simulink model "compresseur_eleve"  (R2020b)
settings: Solver=VariableStepAuto  StartTime=0.0  StopTime=1  RelTol=1e-3
PreLoadFcn:
  | compresseur_7_DataFile
model workspace: external: MATLAB File (data not in the file)
undefined symbols (not defined in the file or in its folder): deg, kg, m, mm, N, s, smiData, X, Y, Z
libraries: sm_lib x91, fl_lib x8, nesl_utility x5, ee_lib x1
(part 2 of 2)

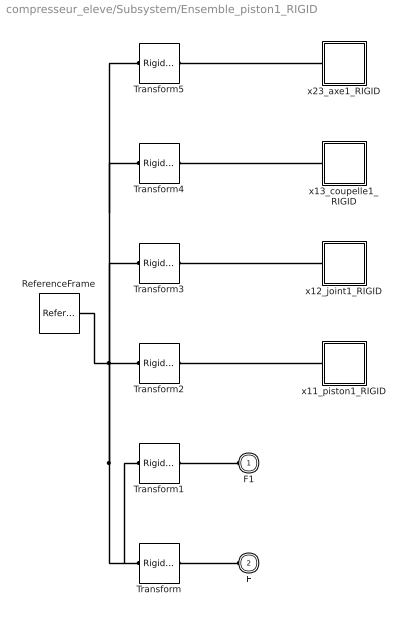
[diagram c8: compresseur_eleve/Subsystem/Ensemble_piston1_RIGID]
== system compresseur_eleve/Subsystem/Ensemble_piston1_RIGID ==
  ReferenceFrame : sm_lib/Frames and Transforms/Reference Frame
  Transform : sm_lib/Frames and Transforms/Rigid Transform  TranslationMethod=Cartesian  TranslationStandardOffset=0  TranslationLengthUnit=mm  TranslationStandardAxis=+Z  TranslationCartesianOffset=smiData.RigidTransform(2).translation  TranslationROffset=0  TranslationROffsetUnits=m  TranslationZOffset=0  TranslationZOffsetUnits=m  TranslationThetaOffset=0  TranslationThetaOffsetUnits=deg  RotationMethod=ArbitraryAxis  RotationAngleUnits=rad  RotationStandardAxis=+Z  RotationAngle=smiData.RigidTransform(2).angle  RotationArbitraryAxis=smiData.RigidTransform(2).axis  FollAlignAxisA=+X  BaseAlignAxisA=+Y  FollAlignAxisB=+Y  BaseAlignAxisB=+Z  RotationSequenceAxes=FollowerAxes  RotationSequence=XYX  RotationSequenceAngles=[0 0 0]  RotationSequenceAnglesUnits=deg  RotationMatrix=[1 0 0; 0 1 0; 0 0 1]
  Transform1 : sm_lib/Frames and Transforms/Rigid Transform  TranslationMethod=Cartesian  TranslationStandardOffset=0  TranslationLengthUnit=mm  TranslationStandardAxis=+Z  TranslationCartesianOffset=smiData.RigidTransform(6).translation  TranslationROffset=0  TranslationROffsetUnits=m  TranslationZOffset=0  TranslationZOffsetUnits=m  TranslationThetaOffset=0  TranslationThetaOffsetUnits=deg  RotationMethod=ArbitraryAxis  RotationAngleUnits=rad  RotationStandardAxis=+Z  RotationAngle=smiData.RigidTransform(6).angle  RotationArbitraryAxis=smiData.RigidTransform(6).axis  FollAlignAxisA=+X  BaseAlignAxisA=+Y  FollAlignAxisB=+Y  BaseAlignAxisB=+Z  RotationSequenceAxes=FollowerAxes  RotationSequence=XYX  RotationSequenceAngles=[0 0 0]  RotationSequenceAnglesUnits=deg  RotationMatrix=[1 0 0; 0 1 0; 0 0 1]
  Transform2 : sm_lib/Frames and Transforms/Rigid Transform  TranslationMethod=Cartesian  TranslationStandardOffset=0  TranslationLengthUnit=mm  TranslationStandardAxis=+Z  TranslationCartesianOffset=smiData.RigidTransform(21).translation  TranslationROffset=0  TranslationROffsetUnits=m  TranslationZOffset=0  TranslationZOffsetUnits=m  TranslationThetaOffset=0  TranslationThetaOffsetUnits=deg  RotationMethod=ArbitraryAxis  RotationAngleUnits=rad  RotationStandardAxis=+Z  RotationAngle=smiData.RigidTransform(21).angle  RotationArbitraryAxis=smiData.RigidTransform(21).axis  FollAlignAxisA=+X  BaseAlignAxisA=+Y  FollAlignAxisB=+Y  BaseAlignAxisB=+Z  RotationSequenceAxes=FollowerAxes  RotationSequence=XYX  RotationSequenceAngles=[0 0 0]  RotationSequenceAnglesUnits=deg  RotationMatrix=[1 0 0; 0 1 0; 0 0 1]
  Transform3 : sm_lib/Frames and Transforms/Rigid Transform  TranslationMethod=Cartesian  TranslationStandardOffset=0  TranslationLengthUnit=mm  TranslationStandardAxis=+Z  TranslationCartesianOffset=smiData.RigidTransform(22).translation  TranslationROffset=0  TranslationROffsetUnits=m  TranslationZOffset=0  TranslationZOffsetUnits=m  TranslationThetaOffset=0  TranslationThetaOffsetUnits=deg  RotationMethod=ArbitraryAxis  RotationAngleUnits=rad  RotationStandardAxis=+Z  RotationAngle=smiData.RigidTransform(22).angle  RotationArbitraryAxis=smiData.RigidTransform(22).axis  FollAlignAxisA=+X  BaseAlignAxisA=+Y  FollAlignAxisB=+Y  BaseAlignAxisB=+Z  RotationSequenceAxes=FollowerAxes  RotationSequence=XYX  RotationSequenceAngles=[0 0 0]  RotationSequenceAnglesUnits=deg  RotationMatrix=[1 0 0; 0 1 0; 0 0 1]
  Transform4 : sm_lib/Frames and Transforms/Rigid Transform  TranslationMethod=Cartesian  TranslationStandardOffset=0  TranslationLengthUnit=mm  TranslationStandardAxis=+Z  TranslationCartesianOffset=smiData.RigidTransform(23).translation  TranslationROffset=0  TranslationROffsetUnits=m  TranslationZOffset=0  TranslationZOffsetUnits=m  TranslationThetaOffset=0  TranslationThetaOffsetUnits=deg  RotationMethod=ArbitraryAxis  RotationAngleUnits=rad  RotationStandardAxis=+Z  RotationAngle=smiData.RigidTransform(23).angle  RotationArbitraryAxis=smiData.RigidTransform(23).axis  FollAlignAxisA=+X  BaseAlignAxisA=+Y  FollAlignAxisB=+Y  BaseAlignAxisB=+Z  RotationSequenceAxes=FollowerAxes  RotationSequence=XYX  RotationSequenceAngles=[0 0 0]  RotationSequenceAnglesUnits=deg  RotationMatrix=[1 0 0; 0 1 0; 0 0 1]
  Transform5 : sm_lib/Frames and Transforms/Rigid Transform  TranslationMethod=Cartesian  TranslationStandardOffset=0  TranslationLengthUnit=mm  TranslationStandardAxis=+Z  TranslationCartesianOffset=smiData.RigidTransform(24).translation  TranslationROffset=0  TranslationROffsetUnits=m  TranslationZOffset=0  TranslationZOffsetUnits=m  TranslationThetaOffset=0  TranslationThetaOffsetUnits=deg  RotationMethod=ArbitraryAxis  RotationAngleUnits=rad  RotationStandardAxis=+Z  RotationAngle=smiData.RigidTransform(24).angle  RotationArbitraryAxis=smiData.RigidTransform(24).axis  FollAlignAxisA=+X  BaseAlignAxisA=+Y  FollAlignAxisB=+Y  BaseAlignAxisB=+Z  RotationSequenceAxes=FollowerAxes  RotationSequence=XYX  RotationSequenceAngles=[0 0 0]  RotationSequenceAnglesUnits=deg  RotationMatrix=[1 0 0; 0 1 0; 0 0 1]
  x11_piston1_RIGID : Subsystem
  x12_joint1_RIGID : Subsystem
  x13_coupelle1_RIGID : Subsystem
  x23_axe1_RIGID : Subsystem
  F1 : PMIOPort  Side=Left
  F : PMIOPort  Port=2  Side=Left
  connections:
  Transform/LConn1 -- ReferenceFrame/RConn1 -- Transform4/LConn1 -- Transform5/LConn1 -- Transform3/LConn1 -- Transform2/LConn1 -- Transform1/LConn1
  Transform/RConn1 -- F/RConn1
  Transform1/RConn1 -- F1/RConn1
  Transform2/RConn1 -- x11_piston1_RIGID/LConn1
  Transform3/RConn1 -- x12_joint1_RIGID/LConn1
  Transform4/RConn1 -- x13_coupelle1_RIGID/LConn1
  Transform5/RConn1 -- x23_axe1_RIGID/LConn1

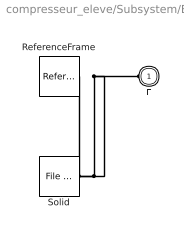
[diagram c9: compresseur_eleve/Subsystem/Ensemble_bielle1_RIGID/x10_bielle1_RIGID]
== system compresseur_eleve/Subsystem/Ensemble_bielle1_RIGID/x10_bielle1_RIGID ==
  ReferenceFrame : sm_lib/Frames and Transforms/Reference Frame
  Solid : sm_lib/Body Elements/File Solid  ExtGeomFileName=10_bielle_ipt_a8871c2b.STL  UnitType=Custom  ExtGeomFileUnits=mm  StepReaderType=HEX  ExportConvexHullGeometry=off  InertiaType=Custom  Mass=smiData.Solid(10).mass  MassUnits=kg  CenterOfMass=smiData.Solid(10).CoM  CenterOfMassUnits=mm  MomentsOfInertia=smiData.Solid(10).MoI  MomentsOfInertiaUnits=kg*mm^2  ProductsOfInertia=smiData.Solid(10).PoI  ProductsOfInertiaUnits=kg*mm^2  BasedOnType=DensityFromFile  Density=1000  DensityUnits=kg/m^3  DoExposeReferenceFrame=on  SerializedFrames=<Frames/>  GraphicType=FromGeometry  MarkerShape=Sphere  MarkerSize=10  GraphicVisPropType=SimpleVisualProperties  GraphicDiffuseColor=smiData.Solid(10).color  GraphicSpecularColor=[0.5 0.5 0.5 1.0]  GraphicAmbientColor=[0.15 0.15 0.15 1.0]  GraphicEmissiveColor=[0.0 0.0 0.0 1.0]  GraphicShininess=75  GraphicOpacity=smiData.Solid(10).opacity
  F : PMIOPort  Side=Left
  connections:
  Solid/RConn1 -- ReferenceFrame/RConn1 -- F/RConn1

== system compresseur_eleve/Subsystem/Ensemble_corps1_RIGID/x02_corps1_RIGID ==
  ReferenceFrame : sm_lib/Frames and Transforms/Reference Frame
  Solid : sm_lib/Body Elements/File Solid  ExtGeomFileName=02_corps_1_ipt_c583bf0c.STL  UnitType=Custom  ExtGeomFileUnits=mm  StepReaderType=HEX  ExportConvexHullGeometry=off  InertiaType=Custom  Mass=smiData.Solid(1).mass  MassUnits=kg  CenterOfMass=smiData.Solid(1).CoM  CenterOfMassUnits=mm  MomentsOfInertia=smiData.Solid(1).MoI  MomentsOfInertiaUnits=kg*mm^2  ProductsOfInertia=smiData.Solid(1).PoI  ProductsOfInertiaUnits=kg*mm^2  BasedOnType=DensityFromFile  Density=1000  DensityUnits=kg/m^3  DoExposeReferenceFrame=on  SerializedFrames=<Frames/>  GraphicType=FromGeometry  MarkerShape=Sphere  MarkerSize=10  GraphicVisPropType=SimpleVisualProperties  GraphicDiffuseColor=smiData.Solid(1).color  GraphicSpecularColor=[0.5 0.5 0.5 1.0]  GraphicAmbientColor=[0.15 0.15 0.15 1.0]  GraphicEmissiveColor=[0.0 0.0 0.0 1.0]  GraphicShininess=75  GraphicOpacity=smiData.Solid(1).opacity
  F : PMIOPort  Side=Left
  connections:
  Solid/RConn1 -- ReferenceFrame/RConn1 -- F/RConn1

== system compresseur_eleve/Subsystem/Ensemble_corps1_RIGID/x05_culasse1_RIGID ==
  ReferenceFrame : sm_lib/Frames and Transforms/Reference Frame
  Solid : sm_lib/Body Elements/File Solid  ExtGeomFileName=05_culasse_1_ipt_d9f37117.STL  UnitType=Custom  ExtGeomFileUnits=mm  StepReaderType=HEX  ExportConvexHullGeometry=off  InertiaType=Custom  Mass=smiData.Solid(2).mass  MassUnits=kg  CenterOfMass=smiData.Solid(2).CoM  CenterOfMassUnits=mm  MomentsOfInertia=smiData.Solid(2).MoI  MomentsOfInertiaUnits=kg*mm^2  ProductsOfInertia=smiData.Solid(2).PoI  ProductsOfInertiaUnits=kg*mm^2  BasedOnType=DensityFromFile  Density=1000  DensityUnits=kg/m^3  DoExposeReferenceFrame=on  SerializedFrames=<Frames/>  GraphicType=FromGeometry  MarkerShape=Sphere  MarkerSize=10  GraphicVisPropType=SimpleVisualProperties  GraphicDiffuseColor=smiData.Solid(2).color  GraphicSpecularColor=[0.5 0.5 0.5 1.0]  GraphicAmbientColor=[0.15 0.15 0.15 1.0]  GraphicEmissiveColor=[0.0 0.0 0.0 1.0]  GraphicShininess=75  GraphicOpacity=smiData.Solid(2).opacity
  F : PMIOPort  Side=Left
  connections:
  Solid/RConn1 -- ReferenceFrame/RConn1 -- F/RConn1

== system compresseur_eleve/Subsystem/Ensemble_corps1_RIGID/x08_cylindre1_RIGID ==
  ReferenceFrame : sm_lib/Frames and Transforms/Reference Frame
  Solid : sm_lib/Body Elements/File Solid  ExtGeomFileName=08_cylindre_1_ipt_a42fec77.STL  UnitType=Custom  ExtGeomFileUnits=mm  StepReaderType=HEX  ExportConvexHullGeometry=off  InertiaType=Custom  Mass=smiData.Solid(3).mass  MassUnits=kg  CenterOfMass=smiData.Solid(3).CoM  CenterOfMassUnits=mm  MomentsOfInertia=smiData.Solid(3).MoI  MomentsOfInertiaUnits=kg*mm^2  ProductsOfInertia=smiData.Solid(3).PoI  ProductsOfInertiaUnits=kg*mm^2  BasedOnType=DensityFromFile  Density=1000  DensityUnits=kg/m^3  DoExposeReferenceFrame=on  SerializedFrames=<Frames/>  GraphicType=FromGeometry  MarkerShape=Sphere  MarkerSize=10  GraphicVisPropType=SimpleVisualProperties  GraphicDiffuseColor=smiData.Solid(3).color  GraphicSpecularColor=[0.5 0.5 0.5 1.0]  GraphicAmbientColor=[0.15 0.15 0.15 1.0]  GraphicEmissiveColor=[0.0 0.0 0.0 1.0]  GraphicShininess=75  GraphicOpacity=smiData.Solid(3).opacity
  F : PMIOPort  Side=Left
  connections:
  Solid/RConn1 -- ReferenceFrame/RConn1 -- F/RConn1

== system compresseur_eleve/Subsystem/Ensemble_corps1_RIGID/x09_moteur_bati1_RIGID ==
  ReferenceFrame : sm_lib/Frames and Transforms/Reference Frame
  Solid : sm_lib/Body Elements/File Solid  ExtGeomFileName=09_moteur_bati_1_ipt_87beb56e.STL  UnitType=Custom  ExtGeomFileUnits=mm  StepReaderType=HEX  ExportConvexHullGeometry=off  InertiaType=Custom  Mass=smiData.Solid(4).mass  MassUnits=kg  CenterOfMass=smiData.Solid(4).CoM  CenterOfMassUnits=mm  MomentsOfInertia=smiData.Solid(4).MoI  MomentsOfInertiaUnits=kg*mm^2  ProductsOfInertia=smiData.Solid(4).PoI  ProductsOfInertiaUnits=kg*mm^2  BasedOnType=DensityFromFile  Density=1000  DensityUnits=kg/m^3  DoExposeReferenceFrame=on  SerializedFrames=<Frames/>  GraphicType=FromGeometry  MarkerShape=Sphere  MarkerSize=10  GraphicVisPropType=SimpleVisualProperties  GraphicDiffuseColor=smiData.Solid(4).color  GraphicSpecularColor=[0.5 0.5 0.5 1.0]  GraphicAmbientColor=[0.15 0.15 0.15 1.0]  GraphicEmissiveColor=[0.0 0.0 0.0 1.0]  GraphicShininess=75  GraphicOpacity=smiData.Solid(4).opacity
  F : PMIOPort  Side=Left
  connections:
  Solid/RConn1 -- ReferenceFrame/RConn1 -- F/RConn1

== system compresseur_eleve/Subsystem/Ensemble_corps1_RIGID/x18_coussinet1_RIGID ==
  ReferenceFrame : sm_lib/Frames and Transforms/Reference Frame
  Solid : sm_lib/Body Elements/File Solid  ExtGeomFileName=18_coussinet_1_ipt_47bc357b.STL  UnitType=Custom  ExtGeomFileUnits=mm  StepReaderType=HEX  ExportConvexHullGeometry=off  InertiaType=Custom  Mass=smiData.Solid(5).mass  MassUnits=kg  CenterOfMass=smiData.Solid(5).CoM  CenterOfMassUnits=mm  MomentsOfInertia=smiData.Solid(5).MoI  MomentsOfInertiaUnits=kg*mm^2  ProductsOfInertia=smiData.Solid(5).PoI  ProductsOfInertiaUnits=kg*mm^2  BasedOnType=DensityFromFile  Density=1000  DensityUnits=kg/m^3  DoExposeReferenceFrame=on  SerializedFrames=<Frames/>  GraphicType=FromGeometry  MarkerShape=Sphere  MarkerSize=10  GraphicVisPropType=SimpleVisualProperties  GraphicDiffuseColor=smiData.Solid(5).color  GraphicSpecularColor=[0.5 0.5 0.5 1.0]  GraphicAmbientColor=[0.15 0.15 0.15 1.0]  GraphicEmissiveColor=[0.0 0.0 0.0 1.0]  GraphicShininess=75  GraphicOpacity=smiData.Solid(5).opacity
  F : PMIOPort  Side=Left
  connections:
  Solid/RConn1 -- ReferenceFrame/RConn1 -- F/RConn1

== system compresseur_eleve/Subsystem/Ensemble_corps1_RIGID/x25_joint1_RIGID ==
  ReferenceFrame : sm_lib/Frames and Transforms/Reference Frame
  Solid : sm_lib/Body Elements/File Solid  ExtGeomFileName=25_joint_1_ipt_2419a34a.STL  UnitType=Custom  ExtGeomFileUnits=mm  StepReaderType=HEX  ExportConvexHullGeometry=off  InertiaType=Custom  Mass=smiData.Solid(6).mass  MassUnits=kg  CenterOfMass=smiData.Solid(6).CoM  CenterOfMassUnits=mm  MomentsOfInertia=smiData.Solid(6).MoI  MomentsOfInertiaUnits=kg*mm^2  ProductsOfInertia=smiData.Solid(6).PoI  ProductsOfInertiaUnits=kg*mm^2  BasedOnType=DensityFromFile  Density=1000  DensityUnits=kg/m^3  DoExposeReferenceFrame=on  SerializedFrames=<Frames/>  GraphicType=FromGeometry  MarkerShape=Sphere  MarkerSize=10  GraphicVisPropType=SimpleVisualProperties  GraphicDiffuseColor=smiData.Solid(6).color  GraphicSpecularColor=[0.5 0.5 0.5 1.0]  GraphicAmbientColor=[0.15 0.15 0.15 1.0]  GraphicEmissiveColor=[0.0 0.0 0.0 1.0]  GraphicShininess=75  GraphicOpacity=smiData.Solid(6).opacity
  F : PMIOPort  Side=Left
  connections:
  Solid/RConn1 -- ReferenceFrame/RConn1 -- F/RConn1

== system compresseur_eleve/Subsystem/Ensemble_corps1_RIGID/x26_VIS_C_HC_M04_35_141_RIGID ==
  ReferenceFrame : sm_lib/Frames and Transforms/Reference Frame
  Solid : sm_lib/Body Elements/File Solid  ExtGeomFileName=26_VIS C HC_ M04-35-14_1_ipt_1f7a07f4.STL  UnitType=Custom  ExtGeomFileUnits=mm  StepReaderType=HEX  ExportConvexHullGeometry=off  InertiaType=Custom  Mass=smiData.Solid(7).mass  MassUnits=kg  CenterOfMass=smiData.Solid(7).CoM  CenterOfMassUnits=mm  MomentsOfInertia=smiData.Solid(7).MoI  MomentsOfInertiaUnits=kg*mm^2  ProductsOfInertia=smiData.Solid(7).PoI  ProductsOfInertiaUnits=kg*mm^2  BasedOnType=DensityFromFile  Density=1000  DensityUnits=kg/m^3  DoExposeReferenceFrame=on  SerializedFrames=<Frames/>  GraphicType=FromGeometry  MarkerShape=Sphere  MarkerSize=10  GraphicVisPropType=SimpleVisualProperties  GraphicDiffuseColor=smiData.Solid(7).color  GraphicSpecularColor=[0.5 0.5 0.5 1.0]  GraphicAmbientColor=[0.15 0.15 0.15 1.0]  GraphicEmissiveColor=[0.0 0.0 0.0 1.0]  GraphicShininess=75  GraphicOpacity=smiData.Solid(7).opacity
  F : PMIOPort  Side=Left
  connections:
  Solid/RConn1 -- ReferenceFrame/RConn1 -- F/RConn1

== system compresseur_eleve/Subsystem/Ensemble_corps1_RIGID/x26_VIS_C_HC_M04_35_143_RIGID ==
  ReferenceFrame : sm_lib/Frames and Transforms/Reference Frame
  Solid : sm_lib/Body Elements/File Solid  ExtGeomFileName=26_VIS C HC_ M04-35-14_ipt_c4dcb1c0.STL  UnitType=Custom  ExtGeomFileUnits=mm  StepReaderType=HEX  ExportConvexHullGeometry=off  InertiaType=Custom  Mass=smiData.Solid(8).mass  MassUnits=kg  CenterOfMass=smiData.Solid(8).CoM  CenterOfMassUnits=mm  MomentsOfInertia=smiData.Solid(8).MoI  MomentsOfInertiaUnits=kg*mm^2  ProductsOfInertia=smiData.Solid(8).PoI  ProductsOfInertiaUnits=kg*mm^2  BasedOnType=DensityFromFile  Density=1000  DensityUnits=kg/m^3  DoExposeReferenceFrame=on  SerializedFrames=<Frames/>  GraphicType=FromGeometry  MarkerShape=Sphere  MarkerSize=10  GraphicVisPropType=SimpleVisualProperties  GraphicDiffuseColor=smiData.Solid(8).color  GraphicSpecularColor=[0.5 0.5 0.5 1.0]  GraphicAmbientColor=[0.15 0.15 0.15 1.0]  GraphicEmissiveColor=[0.0 0.0 0.0 1.0]  GraphicShininess=75  GraphicOpacity=smiData.Solid(8).opacity
  F : PMIOPort  Side=Left
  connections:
  Solid/RConn1 -- ReferenceFrame/RConn1 -- F/RConn1

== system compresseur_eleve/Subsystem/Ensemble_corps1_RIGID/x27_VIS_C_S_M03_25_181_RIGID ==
  ReferenceFrame : sm_lib/Frames and Transforms/Reference Frame
  Solid : sm_lib/Body Elements/File Solid  ExtGeomFileName=27_VIS C S_ M03-25-18_ipt_43eec25f.STL  UnitType=Custom  ExtGeomFileUnits=mm  StepReaderType=HEX  ExportConvexHullGeometry=off  InertiaType=Custom  Mass=smiData.Solid(9).mass  MassUnits=kg  CenterOfMass=smiData.Solid(9).CoM  CenterOfMassUnits=mm  MomentsOfInertia=smiData.Solid(9).MoI  MomentsOfInertiaUnits=kg*mm^2  ProductsOfInertia=smiData.Solid(9).PoI  ProductsOfInertiaUnits=kg*mm^2  BasedOnType=DensityFromFile  Density=1000  DensityUnits=kg/m^3  DoExposeReferenceFrame=on  SerializedFrames=<Frames/>  GraphicType=FromGeometry  MarkerShape=Sphere  MarkerSize=10  GraphicVisPropType=SimpleVisualProperties  GraphicDiffuseColor=smiData.Solid(9).color  GraphicSpecularColor=[0.5 0.5 0.5 1.0]  GraphicAmbientColor=[0.15 0.15 0.15 1.0]  GraphicEmissiveColor=[0.0 0.0 0.0 1.0]  GraphicShininess=75  GraphicOpacity=smiData.Solid(9).opacity
  F : PMIOPort  Side=Left
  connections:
  Solid/RConn1 -- ReferenceFrame/RConn1 -- F/RConn1

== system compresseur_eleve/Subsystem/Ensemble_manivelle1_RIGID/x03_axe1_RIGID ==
  ReferenceFrame : sm_lib/Frames and Transforms/Reference Frame
  Solid : sm_lib/Body Elements/File Solid  ExtGeomFileName=03_axe_ipt_3151f0da.STL  UnitType=Custom  ExtGeomFileUnits=mm  StepReaderType=HEX  ExportConvexHullGeometry=off  InertiaType=Custom  Mass=smiData.Solid(15).mass  MassUnits=kg  CenterOfMass=smiData.Solid(15).CoM  CenterOfMassUnits=mm  MomentsOfInertia=smiData.Solid(15).MoI  MomentsOfInertiaUnits=kg*mm^2  ProductsOfInertia=smiData.Solid(15).PoI  ProductsOfInertiaUnits=kg*mm^2  BasedOnType=DensityFromFile  Density=1000  DensityUnits=kg/m^3  DoExposeReferenceFrame=on  SerializedFrames=<Frames/>  GraphicType=FromGeometry  MarkerShape=Sphere  MarkerSize=10  GraphicVisPropType=SimpleVisualProperties  GraphicDiffuseColor=smiData.Solid(15).color  GraphicSpecularColor=[0.5 0.5 0.5 1.0]  GraphicAmbientColor=[0.15 0.15 0.15 1.0]  GraphicEmissiveColor=[0.0 0.0 0.0 1.0]  GraphicShininess=75  GraphicOpacity=smiData.Solid(15).opacity
  F : PMIOPort  Side=Left
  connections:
  Solid/RConn1 -- ReferenceFrame/RConn1 -- F/RConn1

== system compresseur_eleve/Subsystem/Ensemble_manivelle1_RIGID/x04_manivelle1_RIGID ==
  ReferenceFrame : sm_lib/Frames and Transforms/Reference Frame
  Solid : sm_lib/Body Elements/File Solid  ExtGeomFileName=04_manivelle_ipt_16c0bde3.STL  UnitType=Custom  ExtGeomFileUnits=mm  StepReaderType=HEX  ExportConvexHullGeometry=off  InertiaType=Custom  Mass=smiData.Solid(16).mass  MassUnits=kg  CenterOfMass=smiData.Solid(16).CoM  CenterOfMassUnits=mm  MomentsOfInertia=smiData.Solid(16).MoI  MomentsOfInertiaUnits=kg*mm^2  ProductsOfInertia=smiData.Solid(16).PoI  ProductsOfInertiaUnits=kg*mm^2  BasedOnType=DensityFromFile  Density=1000  DensityUnits=kg/m^3  DoExposeReferenceFrame=on  SerializedFrames=<Frames/>  GraphicType=FromGeometry  MarkerShape=Sphere  MarkerSize=10  GraphicVisPropType=SimpleVisualProperties  GraphicDiffuseColor=smiData.Solid(16).color  GraphicSpecularColor=[0.5 0.5 0.5 1.0]  GraphicAmbientColor=[0.15 0.15 0.15 1.0]  GraphicEmissiveColor=[0.0 0.0 0.0 1.0]  GraphicShininess=75  GraphicOpacity=smiData.Solid(16).opacity
  F : PMIOPort  Side=Left
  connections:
  Solid/RConn1 -- ReferenceFrame/RConn1 -- F/RConn1

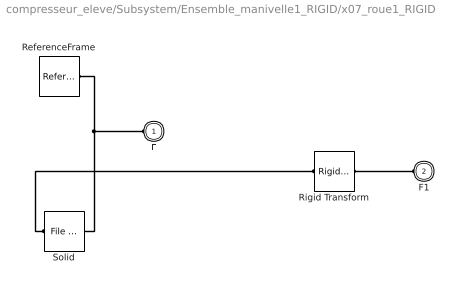
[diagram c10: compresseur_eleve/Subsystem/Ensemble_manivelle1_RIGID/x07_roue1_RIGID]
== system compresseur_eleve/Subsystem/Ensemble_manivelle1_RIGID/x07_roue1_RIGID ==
  ReferenceFrame : sm_lib/Frames and Transforms/Reference Frame
  Rigid Transform : sm_lib/Frames and Transforms/Rigid Transform  TranslationMethod=Cartesian  TranslationStandardOffset=0  TranslationLengthUnit=mm  TranslationStandardAxis=+Z  TranslationCartesianOffset=[0 0 -8]  TranslationROffset=0  TranslationROffsetUnits=m  TranslationZOffset=0  TranslationZOffsetUnits=m  TranslationThetaOffset=0  TranslationThetaOffsetUnits=deg  RotationMethod=None  RotationAngleUnits=deg  RotationStandardAxis=+Z  RotationAngle=0.0  RotationArbitraryAxis=[0 0 1]  FollAlignAxisA=+X  BaseAlignAxisA=+Y  FollAlignAxisB=+Y  BaseAlignAxisB=+Z  RotationSequenceAxes=FollowerAxes  RotationSequence=XYX  RotationSequenceAngles=[0 0 0]  RotationSequenceAnglesUnits=deg  RotationMatrix=[1 0 0; 0 1 0; 0 0 1]
  Solid : sm_lib/Body Elements/File Solid  ExtGeomFileName=07_roue_ipt_2ddf42d4.STL  UnitType=Custom  ExtGeomFileUnits=mm  StepReaderType=HEX  ExportConvexHullGeometry=off  InertiaType=Custom  Mass=smiData.Solid(17).mass  MassUnits=kg  CenterOfMass=smiData.Solid(17).CoM  CenterOfMassUnits=mm  MomentsOfInertia=smiData.Solid(17).MoI  MomentsOfInertiaUnits=kg*mm^2  ProductsOfInertia=smiData.Solid(17).PoI  ProductsOfInertiaUnits=kg*mm^2  BasedOnType=DensityFromFile  Density=1000  DensityUnits=kg/m^3  DoExposeReferenceFrame=on  SerializedFrames=<Frames><Frame><Id>Frame1</Id><Value><Name>F1</Name><Origin><Source>ReferenceFrame</Source><FeatureName></FeatureName></Origin><PrimaryAxis><DefinedDirection>+X</DefinedDirection><Source>CenterOfMassFrame</Source><SourceDirection>-Z</SourceDirection><FeatureName></FeatureName></PrimaryAxis><SecondaryAxis><DefinedDirection>+Z</DefinedDirection><Source>ReferenceFrame</Source><SourceDirection>+X</Sou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  GraphicType=FromGeometry  MarkerShape=Sphere  MarkerSize=10  GraphicVisPropType=SimpleVisualProperties  GraphicDiffuseColor=[0.2 1.0 0.0]  GraphicSpecularColor=[0.5 0.5 0.5 1.0]  GraphicAmbientColor=[0.15 0.15 0.15 1.0]  GraphicEmissiveColor=[0.0 0.0 0.0 1.0]  GraphicShininess=75  GraphicOpacity=smiData.Solid(17).opacity
  F : PMIOPort  Side=Left
  F1 : PMIOPort  Port=2  Side=Left
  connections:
  ReferenceFrame/RConn1 -- Solid/RConn1 -- F/RConn1
  F1/RConn1 -- Rigid Transform/RConn1
  Solid/LConn1 -- Rigid Transform/LConn1

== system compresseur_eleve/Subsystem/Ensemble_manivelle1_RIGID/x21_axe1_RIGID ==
  ReferenceFrame : sm_lib/Frames and Transforms/Reference Frame
  Solid : sm_lib/Body Elements/File Solid  ExtGeomFileName=21_axe_ipt_8876eebc.STL  UnitType=Custom  ExtGeomFileUnits=mm  StepReaderType=HEX  ExportConvexHullGeometry=off  InertiaType=Custom  Mass=smiData.Solid(18).mass  MassUnits=kg  CenterOfMass=smiData.Solid(18).CoM  CenterOfMassUnits=mm  MomentsOfInertia=smiData.Solid(18).MoI  MomentsOfInertiaUnits=kg*mm^2  ProductsOfInertia=smiData.Solid(18).PoI  ProductsOfInertiaUnits=kg*mm^2  BasedOnType=DensityFromFile  Density=1000  DensityUnits=kg/m^3  DoExposeReferenceFrame=on  SerializedFrames=<Frames/>  GraphicType=FromGeometry  MarkerShape=Sphere  MarkerSize=10  GraphicVisPropType=SimpleVisualProperties  GraphicDiffuseColor=smiData.Solid(18).color  GraphicSpecularColor=[0.5 0.5 0.5 1.0]  GraphicAmbientColor=[0.15 0.15 0.15 1.0]  GraphicEmissiveColor=[0.0 0.0 0.0 1.0]  GraphicShininess=75  GraphicOpacity=smiData.Solid(18).opacity
  F : PMIOPort  Side=Left
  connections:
  Solid/RConn1 -- ReferenceFrame/RConn1 -- F/RConn1

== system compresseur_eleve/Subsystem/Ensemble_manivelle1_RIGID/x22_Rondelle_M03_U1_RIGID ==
  ReferenceFrame : sm_lib/Frames and Transforms/Reference Frame
  Solid : sm_lib/Body Elements/File Solid  ExtGeomFileName=22_Rondelle M03 U_ipt_6859df5.STL  UnitType=Custom  ExtGeomFileUnits=mm  StepReaderType=HEX  ExportConvexHullGeometry=off  InertiaType=Custom  Mass=smiData.Solid(19).mass  MassUnits=kg  CenterOfMass=smiData.Solid(19).CoM  CenterOfMassUnits=mm  MomentsOfInertia=smiData.Solid(19).MoI  MomentsOfInertiaUnits=kg*mm^2  ProductsOfInertia=smiData.Solid(19).PoI  ProductsOfInertiaUnits=kg*mm^2  BasedOnType=DensityFromFile  Density=1000  DensityUnits=kg/m^3  DoExposeReferenceFrame=on  SerializedFrames=<Frames/>  GraphicType=FromGeometry  MarkerShape=Sphere  MarkerSize=10  GraphicVisPropType=SimpleVisualProperties  GraphicDiffuseColor=smiData.Solid(19).color  GraphicSpecularColor=[0.5 0.5 0.5 1.0]  GraphicAmbientColor=[0.15 0.15 0.15 1.0]  GraphicEmissiveColor=[0.0 0.0 0.0 1.0]  GraphicShininess=75  GraphicOpacity=smiData.Solid(19).opacity
  F : PMIOPort  Side=Left
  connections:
  Solid/RConn1 -- ReferenceFrame/RConn1 -- F/RConn1

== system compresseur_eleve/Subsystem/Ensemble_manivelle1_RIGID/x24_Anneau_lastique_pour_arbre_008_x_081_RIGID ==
  ReferenceFrame : sm_lib/Frames and Transforms/Reference Frame
  Solid : sm_lib/Body Elements/File Solid  ExtGeomFileName=24_Anneau élastique pour arbre_ 008 x 08_ipt_949c560f.STL  UnitType=Custom  ExtGeomFileUnits=mm  StepReaderType=HEX  ExportConvexHullGeometry=off  InertiaType=Custom  Mass=smiData.Solid(20).mass  MassUnits=kg  CenterOfMass=smiData.Solid(20).CoM  CenterOfMassUnits=mm  MomentsOfInertia=smiData.Solid(20).MoI  MomentsOfInertiaUnits=kg*mm^2  ProductsOfInertia=smiData.Solid(20).PoI  ProductsOfInertiaUnits=kg*mm^2  BasedOnType=DensityFromFile  Density=1000  DensityUnits=kg/m^3  DoExposeReferenceFrame=on  SerializedFrames=<Frames/>  GraphicType=FromGeometry  MarkerShape=Sphere  MarkerSize=10  GraphicVisPropType=SimpleVisualProperties  GraphicDiffuseColor=smiData.Solid(20).color  GraphicSpecularColor=[0.5 0.5 0.5 1.0]  GraphicAmbientColor=[0.15 0.15 0.15 1.0]  GraphicEmissiveColor=[0.0 0.0 0.0 1.0]  GraphicShininess=75  GraphicOpacity=smiData.Solid(20).opacity
  F : PMIOPort  Side=Left
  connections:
  Solid/RConn1 -- ReferenceFrame/RConn1 -- F/RConn1

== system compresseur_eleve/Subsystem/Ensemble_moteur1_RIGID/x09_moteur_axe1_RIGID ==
  ReferenceFrame : sm_lib/Frames and Transforms/Reference Frame
  Solid : sm_lib/Body Elements/File Solid  ExtGeomFileName=09_moteur_axe_ipt_20b3807d.STL  UnitType=Custom  ExtGeomFileUnits=mm  StepReaderType=HEX  ExportConvexHullGeometry=off  InertiaType=Custom  Mass=smiData.Solid(21).mass  MassUnits=kg  CenterOfMass=smiData.Solid(21).CoM  CenterOfMassUnits=mm  MomentsOfInertia=smiData.Solid(21).MoI  MomentsOfInertiaUnits=kg*mm^2  ProductsOfInertia=smiData.Solid(21).PoI  ProductsOfInertiaUnits=kg*mm^2  BasedOnType=DensityFromFile  Density=1000  DensityUnits=kg/m^3  DoExposeReferenceFrame=on  SerializedFrames=<Frames/>  GraphicType=FromGeometry  MarkerShape=Sphere  MarkerSize=10  GraphicVisPropType=SimpleVisualProperties  GraphicDiffuseColor=smiData.Solid(21).color  GraphicSpecularColor=[0.5 0.5 0.5 1.0]  GraphicAmbientColor=[0.15 0.15 0.15 1.0]  GraphicEmissiveColor=[0.0 0.0 0.0 1.0]  GraphicShininess=75  GraphicOpacity=smiData.Solid(21).opacity
  F : PMIOPort  Side=Left
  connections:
  Solid/RConn1 -- ReferenceFrame/RConn1 -- F/RConn1

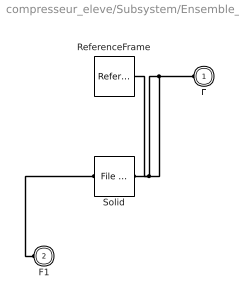
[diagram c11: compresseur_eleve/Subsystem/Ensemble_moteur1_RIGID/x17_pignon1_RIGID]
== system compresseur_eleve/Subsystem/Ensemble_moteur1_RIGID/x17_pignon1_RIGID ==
  ReferenceFrame : sm_lib/Frames and Transforms/Reference Frame
  Solid : sm_lib/Body Elements/File Solid  ExtGeomFileName=17_pignon_ipt_e84d4c85.STL  UnitType=Custom  ExtGeomFileUnits=mm  StepReaderType=HEX  ExportConvexHullGeometry=off  InertiaType=Custom  Mass=smiData.Solid(22).mass  MassUnits=kg  CenterOfMass=smiData.Solid(22).CoM  CenterOfMassUnits=mm  MomentsOfInertia=smiData.Solid(22).MoI  MomentsOfInertiaUnits=kg*mm^2  ProductsOfInertia=smiData.Solid(22).PoI  ProductsOfInertiaUnits=kg*mm^2  BasedOnType=DensityFromFile  Density=1000  DensityUnits=kg/m^3  DoExposeReferenceFrame=on  SerializedFrames=<Frames><Frame><Id>Frame1</Id><Value><Name>F1</Name><Origin><Source>ReferenceFrame</Source><FeatureName></FeatureName></Origin><PrimaryAxis><DefinedDirection>+Z</DefinedDirection><Source>ReferenceFrame</Source><SourceDirection>+Z</SourceDirection><FeatureName></FeatureName></PrimaryAxis><SecondaryAxis><DefinedDirection>+X</DefinedDirection><Source>ReferenceFrame</Source><SourceDirection>+X</Source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  GraphicType=FromGeometry  MarkerShape=Sphere  MarkerSize=10  GraphicVisPropType=SimpleVisualProperties  GraphicDiffuseColor=smiData.Solid(22).color  GraphicSpecularColor=[0.5 0.5 0.5 1.0]  GraphicAmbientColor=[0.15 0.15 0.15 1.0]  GraphicEmissiveColor=[0.0 0.0 0.0 1.0]  GraphicShininess=75  GraphicOpacity=smiData.Solid(22).opacity
  F : PMIOPort  Side=Left
  F1 : PMIOPort  Port=2  Side=Left
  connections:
  Solid/RConn1 -- ReferenceFrame/RConn1 -- F/RConn1
  F1/RConn1 -- Solid/LConn1

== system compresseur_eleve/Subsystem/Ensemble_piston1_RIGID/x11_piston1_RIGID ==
  ReferenceFrame : sm_lib/Frames and Transforms/Reference Frame
  Solid : sm_lib/Body Elements/File Solid  ExtGeomFileName=11_piston_ipt_eda23d89.STL  UnitType=Custom  ExtGeomFileUnits=mm  StepReaderType=HEX  ExportConvexHullGeometry=off  InertiaType=Custom  Mass=smiData.Solid(11).mass  MassUnits=kg  CenterOfMass=smiData.Solid(11).CoM  CenterOfMassUnits=mm  MomentsOfInertia=smiData.Solid(11).MoI  MomentsOfInertiaUnits=kg*mm^2  ProductsOfInertia=smiData.Solid(11).PoI  ProductsOfInertiaUnits=kg*mm^2  BasedOnType=DensityFromFile  Density=1000  DensityUnits=kg/m^3  DoExposeReferenceFrame=on  SerializedFrames=<Frames/>  GraphicType=FromGeometry  MarkerShape=Sphere  MarkerSize=10  GraphicVisPropType=SimpleVisualProperties  GraphicDiffuseColor=smiData.Solid(11).color  GraphicSpecularColor=[0.5 0.5 0.5 1.0]  GraphicAmbientColor=[0.15 0.15 0.15 1.0]  GraphicEmissiveColor=[0.0 0.0 0.0 1.0]  GraphicShininess=75  GraphicOpacity=smiData.Solid(11).opacity
  F : PMIOPort  Side=Left
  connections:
  Solid/RConn1 -- ReferenceFrame/RConn1 -- F/RConn1

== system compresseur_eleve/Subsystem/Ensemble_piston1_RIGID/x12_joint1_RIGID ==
  ReferenceFrame : sm_lib/Frames and Transforms/Reference Frame
  Solid : sm_lib/Body Elements/File Solid  ExtGeomFileName=12_joint_ipt_f9a651d5.STL  UnitType=Custom  ExtGeomFileUnits=mm  StepReaderType=HEX  ExportConvexHullGeometry=off  InertiaType=Custom  Mass=smiData.Solid(12).mass  MassUnits=kg  CenterOfMass=smiData.Solid(12).CoM  CenterOfMassUnits=mm  MomentsOfInertia=smiData.Solid(12).MoI  MomentsOfInertiaUnits=kg*mm^2  ProductsOfInertia=smiData.Solid(12).PoI  ProductsOfInertiaUnits=kg*mm^2  BasedOnType=DensityFromFile  Density=1000  DensityUnits=kg/m^3  DoExposeReferenceFrame=on  SerializedFrames=<Frames/>  GraphicType=FromGeometry  MarkerShape=Sphere  MarkerSize=10  GraphicVisPropType=SimpleVisualProperties  GraphicDiffuseColor=smiData.Solid(12).color  GraphicSpecularColor=[0.5 0.5 0.5 1.0]  GraphicAmbientColor=[0.15 0.15 0.15 1.0]  GraphicEmissiveColor=[0.0 0.0 0.0 1.0]  GraphicShininess=75  GraphicOpacity=smiData.Solid(12).opacity
  F : PMIOPort  Side=Left
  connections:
  Solid/RConn1 -- ReferenceFrame/RConn1 -- F/RConn1

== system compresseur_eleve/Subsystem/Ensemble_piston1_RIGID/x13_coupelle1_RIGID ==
  ReferenceFrame : sm_lib/Frames and Transforms/Reference Frame
  Solid : sm_lib/Body Elements/File Solid  ExtGeomFileName=13_coupelle_ipt_9621d9ed.STL  UnitType=Custom  ExtGeomFileUnits=mm  StepReaderType=HEX  ExportConvexHullGeometry=off  InertiaType=Custom  Mass=smiData.Solid(13).mass  MassUnits=kg  CenterOfMass=smiData.Solid(13).CoM  CenterOfMassUnits=mm  MomentsOfInertia=smiData.Solid(13).MoI  MomentsOfInertiaUnits=kg*mm^2  ProductsOfInertia=smiData.Solid(13).PoI  ProductsOfInertiaUnits=kg*mm^2  BasedOnType=DensityFromFile  Density=1000  DensityUnits=kg/m^3  DoExposeReferenceFrame=on  SerializedFrames=<Frames/>  GraphicType=FromGeometry  MarkerShape=Sphere  MarkerSize=10  GraphicVisPropType=SimpleVisualProperties  GraphicDiffuseColor=smiData.Solid(13).color  GraphicSpecularColor=[0.5 0.5 0.5 1.0]  GraphicAmbientColor=[0.15 0.15 0.15 1.0]  GraphicEmissiveColor=[0.0 0.0 0.0 1.0]  GraphicShininess=75  GraphicOpacity=smiData.Solid(13).opacity
  F : PMIOPort  Side=Left
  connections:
  Solid/RConn1 -- ReferenceFrame/RConn1 -- F/RConn1

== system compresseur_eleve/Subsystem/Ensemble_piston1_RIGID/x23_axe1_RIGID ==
  ReferenceFrame : sm_lib/Frames and Transforms/Reference Frame
  Solid : sm_lib/Body Elements/File Solid  ExtGeomFileName=23_axe_ipt_8876eebc.STL  UnitType=Custom  ExtGeomFileUnits=mm  StepReaderType=HEX  ExportConvexHullGeometry=off  InertiaType=Custom  Mass=smiData.Solid(14).mass  MassUnits=kg  CenterOfMass=smiData.Solid(14).CoM  CenterOfMassUnits=mm  MomentsOfInertia=smiData.Solid(14).MoI  MomentsOfInertiaUnits=kg*mm^2  ProductsOfInertia=smiData.Solid(14).PoI  ProductsOfInertiaUnits=kg*mm^2  BasedOnType=DensityFromFile  Density=1000  DensityUnits=kg/m^3  DoExposeReferenceFrame=on  SerializedFrames=<Frames/>  GraphicType=FromGeometry  MarkerShape=Sphere  MarkerSize=10  GraphicVisPropType=SimpleVisualProperties  GraphicDiffuseColor=smiData.Solid(14).color  GraphicSpecularColor=[0.5 0.5 0.5 1.0]  GraphicAmbientColor=[0.15 0.15 0.15 1.0]  GraphicEmissiveColor=[0.0 0.0 0.0 1.0]  GraphicShininess=75  GraphicOpacity=smiData.Solid(14).opacity
  F : PMIOPort  Side=Left
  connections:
  Solid/RConn1 -- ReferenceFrame/RConn1 -- F/RConn1
